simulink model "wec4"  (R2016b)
settings: Solver=ode4  StartTime=0  StopTime=1000  FixedStep=0.005  MaxStep=0.005  RelTol=1e-3  EnableMultiTasking=on
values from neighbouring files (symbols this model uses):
  arAdaptiveLawData = 1/2*zModelSimple.zModelPto.arFreq.*     zModelSimple.zModelPto.arMagnitude./     cos(zModelSimple.zModelPto.arPhase*pi/180+pi/2)    [IMPACT_Control.m]
  arAdaptiveLawDataX = 1/2*zModelSimpleX.zModelPto.arFreq.*         zModelSimpleX.zModelPto.arMagnitude./         cos(zModelSimpleX.zModelPto.arPhase*pi/180+pi/2)    [IMPACT_Control.m]
  arControllerRampGain = [0,0,1,1]    [IMPACT_Control.m]
  arControllerRampTime = [0 rStartRampTime rStartRampTime+rRampTimeLength 8000]    [IMPACT_Control.m]
  arEkfInitialisation = zeros(1,11)    [IMPACT_Control.m]
  arEkfInitialisationX = zeros(1,11)    [IMPACT_Control.m]
  arFrequency = zModelSimple.zModelPto.arFreq    [IMPACT_Control.m]
  arFrequencyRange = zModelSimple.zModelPto.arFreq    [IMPACT_Control.m]
  arFrequencyX = zModelSimpleX.zModelPto.arFreq    [IMPACT_Control.m]
  arImpedance = 1./zModelSimple.zModelPto.arMagnitude./zModelSimple.zModelPto.arFreq    [IMPACT_Control.m]
  arImpedanceX = 1./zModelSimpleX.zModelPto.arMagnitude./zModelSimpleX.zModelPto.arFreq    [IMPACT_Control.m]
  CentralPTOPreload = -1.6113e+07    (= -16113000)    [wecSimInputFile.m]
  F1 = [4.243 2.375 -12.243]    [wecSimInputFile.m]
  F2 = [4.243 -2.375 -12.243]    [wecSimInputFile.m]
  F3 = [-4.243 -2.375 -12.243]    [wecSimInputFile.m]
  F4 = [-4.243 2.375 -12.243]    [wecSimInputFile.m]
  FC = [0 0 -14]    [wecSimInputFile.m]
  iAdaptiveDamping = 0    [wec4IMPACT_Project.m]    (also in IMPACT_Control.m = handles.iAdaptiveDamping; wec1_IMPACT_Project.m; wec2_IMPACT_Project.m; wec3_IMPACT_Project.m)
  iControlType = 2    [wec4IMPACT_Project.m]    (also in IMPACT_Control.m = handles.iControlType; wec1_IMPACT_Project.m = 1; wec2_IMPACT_Project.m = 1; wec3_IMPACT_Project.m = 1)
  iPtoPositionConstraint = 1    [wec4IMPACT_Project.m]    (also in IMPACT_Control.m = handles.iPtoPositionConstraint; wec1_IMPACT_Project.m = 0; wec2_IMPACT_Project.m; wec3_IMPACT_Project.m)
  iSensorNoise = 0    [IMPACT_Control.m]
  m = m+1    (= 2)    [checkParamFile.m]
  PTOrotation = atan((T1(2)-F1(2))/(T1(1)-F1(1)))    [wecSimInputFile.m]
  rCogFloater = -8    [wec4_IMPACT_Model.m]    (also in paramInitial.m = get( handles.edit_rCogFloater, 'String' ); wec1_IMPACT_Model.m = -18; wec2_IMPACT_Model.m = -8.5; wec3_IMPACT_Model.m = -0.7)
  rCogSpar = -36.6    [wec4_IMPACT_Model.m]    (also in paramInitial.m = get( handles.edit_rCogSpar, 'String' ); wec3_IMPACT_Model.m = -21.3; wec3_IMPACT_Model2.m = -21.3)
  rDisplacementLimit = 10.000000    (= 10)    [wec4IMPACT_Project.m]    (also in IMPACT_Control.m = getValue(handles.edit_displacementLimit); wec1_IMPACT_Project.m; wec2_IMPACT_Project.m; wec3_IMPACT_Project.m = 3)
  rDisplacementLimitX = 10.000000    (= 10)    [wec4IMPACT_Project.m]    (also in IMPACT_Control.m = getValue(handles.edit_displacementLimitX); wec1_IMPACT_Project.m = 0; wec2_IMPACT_Project.m; wec3_IMPACT_Project.m = 0)
  rGainForAntiWIndUp = tfControllerDiscrete.rGain    [IMPACT_Control.m]
  rGainForAntiWIndUpX = tfControllerXDiscrete.rGain    [IMPACT_Control.m]
  rMaxForcePto = 300000000.000000    (= 300000000)    [wec4IMPACT_Project.m]    (also in IMPACT_Control.m = getValue(handles.edit_maxForcePto); wec1_IMPACT_Project.m = 1e+15; wec2_IMPACT_Project.m = 1e+15; wec3_IMPACT_Project.m = 1000000000)
  rMinForcePto = -300000000.000000    (= -300000000)    [wec4IMPACT_Project.m]    (also in IMPACT_Control.m = getValue(handles.edit_minForcePto); wec1_IMPACT_Project.m = -1e+15; wec2_IMPACT_Project.m = -1e+15; wec3_IMPACT_Project.m = -1000000000)
  rMooringX = 20000    [wec4_IMPACT_Model.m]    (also in paramInitial.m = get( handles.edit_rMooringX, 'String' ); wec3_IMPACT_Model.m = 10000; wec3_IMPACT_Model2.m = 10000)
  rMooringZ = 10000    [wec4_IMPACT_Model.m]    (also in paramInitial.m = get( handles.edit_rMooringZ, 'String' ); wec3_IMPACT_Model.m = 0; wec3_IMPACT_Model2.m = 0)
  rOutputSampleTime = 0.010000    (= 0.01)    [wec4IMPACT_Project.m]    (also in IMPACT_Control.m = getValue(handles.edit_outputSampleTime); wec1_IMPACT_Project.m; wec2_IMPACT_Project.m; wec3_IMPACT_Project.m)
  rPassiveDampingGain = -604830.000000    (= -604830)    [wec4IMPACT_Project.m]    (also in IMPACT_Control.m = getValue(handles.edit_gainPLD); wec1_IMPACT_Project.m = -214018.1537; wec2_IMPACT_Project.m = -1948070; wec3_IMPACT_Project.m = -519390)
  rPassiveDampingGainX = -278660.000000    (= -278660)    [wec4IMPACT_Project.m]    (also in IMPACT_Control.m = getValue(handles.edit_gainPLDX); wec1_IMPACT_Project.m = 0; wec2_IMPACT_Project.m = 0; wec3_IMPACT_Project.m = 0)
  rTetherPretension = 1.6113e+07    (= 16113000)    [wec4_IMPACT_Model.m]    (also in paramInitial.m = get( handles.edit_rTetherPretension, 'String' ); wec3_IMPACT_Model.m = 0; wec3_IMPACT_Model2.m = 0)
  rTetherSpring = 500000    [wec4_IMPACT_Model.m]    (also in paramInitial.m = get( handles.edit_rTetherSpring, 'String' ); wec3_IMPACT_Model.m = 0; wec3_IMPACT_Model2.m = 0)
  rUpperFrequencyLimit = EKFFloater.upperFreq    [IMPACT_Control.m]
  rXf = 4.243    [wec4AdditionalParams.m]
  rXs = 16.075    [wec4AdditionalParams.m]
  rYf = 2.375    [wec4AdditionalParams.m]
  rYs = 16.075    [wec4AdditionalParams.m]
  rZf = 4.243    [wec4AdditionalParams.m]
  rZs = 2.4350    (= 2.435)    [wec4AdditionalParams.m]
  rZTetherF = 6    [wec4AdditionalParams.m]
  rZTetherS = 2.4350    (= 2.435)    [wec4AdditionalParams.m]
  s = tf('s')    [wec4_IMPACT_Model.m]    (also in IMPACT_Control.m; wec1_IMPACT_Model.m; wec2_IMPACT_Model.m; wec3_IMPACT_Model.m)
  SidePTO1Preload = PreloadPTOCorner    (= 0)    [wecSimInputFile.m]
  SidePTO2Preload = PreloadPTOCorner    (= 0)    [wecSimInputFile.m]
  SidePTO3Preload = PreloadPTOCorner    (= 0)    [wecSimInputFile.m]
  SidePTO4Preload = PreloadPTOCorner    (= 0)    [wecSimInputFile.m]
  simu = simulationClass()    [wecSimInputFile.m]
  T1 = [16.075 16.075 -34.165]    [wecSimInputFile.m]
  T2 = [16.075 -16.075 -34.165]    [wecSimInputFile.m]
  T3 = [-16.075 -16.075 -34.165]    [wecSimInputFile.m]
  T4 = [-16.075 16.075 -34.165]    [wecSimInputFile.m]
  TC = [0 0 -34.165]    [wecSimInputFile.m]
  waves = waveClass('irregular')    [wecSimInputFile.m]
  Z = magPhaseToComplex(zModelTf)    [IMPACT_Control.m]
undefined symbols (not defined in the file or in its folder): arControllerDiscreteDen, arControllerDiscreteNum, arControllerDiscreteXDen, arControllerDiscreteXNum, arExcForceFloaterDen, arExcForceFloaterNum, arExcForceFloaterXDen, arExcForceFloaterXNum, arExcForceSparDen, arExcForceSparNum, arExcForceSparXDen, arExcForceSparXNum, arFexcFloaterDen, arFexcFloaterNum, arFexcFloaterXDen, arFexcFloaterXNum, arFexcSparDen, arFexcSparNum, arFexcSparXDen, arFexcSparXNum, Body, body, constraint, CTTime, deg, Elements, geometry, IRKB, kg, lenJ, mooring, N, pto, rAccelerationGainFloater, rAccelerationGainFloaterX, rAccelerationGainSpar, rAccelerationGainSparX, rad, rBuoyancyGainFloater, rBuoyancyGainFloaterX, rBuoyancyGainSpar, rBuoyancyGainSparX, rDampingGainFloater, rDampingGainFloaterX, rDampingGainSpar, rDampingGainSparX, Rigid, rMaxFocePto, wec4_float, wec4_reactor, WECSim_Lib, X, Y
libraries: nesl_utility x380, sm_lib x170, vrlib x91, simulink x12, WECSim_Lib x4
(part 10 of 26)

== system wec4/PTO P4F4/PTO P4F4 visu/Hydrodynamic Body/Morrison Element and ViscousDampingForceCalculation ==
  Displacement : Inport
  Acceleration : Inport  Port=2
  Velocity : Inport  Port=3
  Time : Inport  Port=4
  Abs1 : Abs
  Morrison Element Variant Subsystem : Subsystem  Variant=on
  Product : Product
  Product1 : Product  Multiplication=Matrix(*)
  Transport Delay : TransportDelay  DelayTime=10e-8
  "VisSum " : Sum  Inputs=+-
  "Viscous Damping Matrix (diagonal) " : Constant  Value=body.hydroForce.visDrag
  F_MorrisonAndViscous : Outport
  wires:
  Time/1 -> Morrison Element Variant Subsystem/4(time)
  Morrison Element Variant Subsystem/1(morison_force) -> "VisSum "/2
  Displacement/1 -> Morrison Element Variant Subsystem/1(displacement)
  Product/1 -> Product1/2  "v * |v|"
  "Viscous Damping Matrix (diagonal) "/1 -> Product1/1  "0.5 * cd * rho *A"
  Product1/1 -> "VisSum "/1
  Abs1/1 -> Product/2
  Acceleration/1 -> Transport Delay/1
  Transport Delay/1 -> Morrison Element Variant Subsystem/3(acceleration)
  "VisSum "/1 -> F_MorrisonAndViscous/1  "F_MorrisonAndViscous"
  Velocity/1 -> Abs1/1, Product/1, Morrison Element Variant Subsystem/2(velocity)

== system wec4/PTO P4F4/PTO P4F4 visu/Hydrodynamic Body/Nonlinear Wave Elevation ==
  Displacement : Inport
  Time : Inport  Port=2
  Add : Sum  Inputs=+-
  Center of Gravity : Constant  Value=body.cg
  Constant : Constant  Value=[0 0 0]
  Linear or Instantaneous Free Surface : Subsystem  Variant=on
  Mux : Mux  Inputs=2
  Wave Elevation : Outport
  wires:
  Time/1 -> Linear or Instantaneous Free Surface/2(In2)
  Constant/1 -> Mux/2
  Center of Gravity/1 -> Mux/1  "cg"
  Mux/1 -> Add/2
  Add/1 -> Linear or Instantaneous Free Surface/1(In1)  "x_cg"
  Linear or Instantaneous Free Surface/1(Out1) -> Wave Elevation/1
  Displacement/1 -> Add/1  "x"

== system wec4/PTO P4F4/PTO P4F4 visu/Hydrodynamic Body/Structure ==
  Total Force : Inport
  Body Properties : sm_lib/Body Elements/Solid  InertiaType=Custom  Mass=body.mass  MassUnits=kg  CenterOfMass=[0 0 0]  CenterOfMassUnits=m  MomentsOfInertia=body.momOfInertia  MomentsOfInertiaUnits=kg*m^2  ProductsOfInertia=[0 0 0]  ProductsOfInertiaUnits=kg*m^2  DensityBased=on  Density=1000  DensityUnits=kg/(m^3)  DoExposeReferenceFrame=on  SerializedFrames=<Frames/>  GraphicType=FromGeometry  MarkerShape=Sphere  MarkerSize=10  MarkerSizeUnits=m  GraphicVisPropType=SimpleVisualProperties  GraphicDiffuseColor=body.viz.color  GraphicSpecularColor=[0.5 0.5 0.5 1.0]  GraphicAmbientColor=[0.15 0.15 0.15 1.0]  GraphicEmissiveColor=[0.0 0.0 0.0 1.0]  GraphicShininess=75  GraphicOpacity=body.viz.opacity  GeometryShape=FromFile  RectangleSize=[1 1]  RectangleSizeUnits=m  BrickDimensions=[1 1 1]  BrickDimensionUnits=m  CylinderRadius=1  CylinderRadiusUnits=m  CylinderLength=1  CylinderLengthUnits=m  SphereRadius=1  SphereRadiusUnits=m  EllipsoidRadii=[1 1 1]  EllipsoidRadiiUnits=m  ExtrusionCrossSection=[1 1; -1 1; -1 -1; 1 -1]  ExtrusionCrossSectionUnits=m  ExtrusionLength=1  ExtrusionLengthUnits=m  PolygonNumSides=3  PolygonOuterRadius=1  PolygonOuterRadiusUnits=m  ExtGeomFileType=STL  ExtGeomFileName=.\geometry\pto_visu.stl  ExtGeomFileUnits=m  RevolutionCrossSection=[1 1; 1 -1; 2 -1; 2 1]  RevolutionCrossSectionUnits=m  RevolutionExtent=Full  RevolutionAngle=180  RevolutionAngleUnits=deg
  External Force and Torque : sm_lib/Forces and Torques/External Force and Torque  ForceResolutionFrame=World  EnableForceX=off  EnableForceY=off  EnableForceZ=off  EnableForce=on  TorqueResolutionFrame=World  EnableTorqueX=off  EnableTorqueY=off  EnableTorqueZ=off  EnableTorque=on
  Motion Sensor : Subsystem
  Rigid Transform (Setup CG) : sm_lib/Frames and Transforms/Rigid Transform  TranslationMethod=Cartesian  TranslationStandardOffset=0  TranslationLengthUnit=m  TranslationStandardAxis=+Z  TranslationCartesianOffset=body.cg  TranslationROffset=0  TranslationROffsetUnits=m  TranslationZOffset=0  TranslationZOffsetUnits=m  TranslationThetaOffset=0  TranslationThetaOffsetUnits=deg  RotationMethod=None  RotationAngleUnits=rad  RotationStandardAxis=+Y  RotationAngle=0.05  RotationArbitraryAxis=[0.57735026918962584 0.57735026918962584 0.57735026918962584]  FollAlignAxisA=+X  BaseAlignAxisA=+Y  FollAlignAxisB=+Y  BaseAlignAxisB=+Z  RotationSequenceAxes=FollowerAxes  RotationSequence=XYX  RotationSequenceAngles=[0 0 0]  RotationSequenceAnglesUnits=deg  RotationMatrix=[1 0 0; 0 1 0; 0 0 1]
  Rigid Transform (Setup Initial Disp) : sm_lib/Frames and Transforms/Rigid Transform  TranslationMethod=Cartesian  TranslationStandardOffset=0  TranslationLengthUnit=m  TranslationStandardAxis=+Z  TranslationCartesianOffset=body.initDisp.initLinDisp  TranslationROffset=0  TranslationROffsetUnits=m  TranslationZOffset=0  TranslationZOffsetUnits=m  TranslationThetaOffset=0  TranslationThetaOffsetUnits=deg  RotationMethod=ArbitraryAxis  RotationAngleUnits=rad  RotationStandardAxis=+Y  RotationAngle=body.initDisp.initAngularDispAngle  RotationArbitraryAxis=body.initDisp.initAngularDispAxis  FollAlignAxisA=+X  BaseAlignAxisA=+Y  FollAlignAxisB=+Y  BaseAlignAxisB=+Z  RotationSequenceAxes=FollowerAxes  RotationSequence=XYX  RotationSequenceAngles=[0 0 0]  RotationSequenceAnglesUnits=deg  RotationMatrix=[1 0 0; 0 1 0; 0 0 1]
  Selector : Selector  InputPortWidth=6  IndexOptions=Index vector (dialog)  Indices=[1:3]  OutputSizes=1
  Selector1 : Selector  InputPortWidth=6  IndexOptions=Index vector (dialog)  Indices=[4:6]  OutputSizes=1
  Simulink-PS Converter1 : nesl_utility/Simulink-PS Converter  PhysicalDomain=network_engine_domain  SubClassName=ps_input  LeftPortType=input  RightPortType=output  PseudoPeriodic=off  Frequencies=[]  NoiseDistribution=none  NoiseParameters=[]  Unit=1  AffineConversion=off  InputFiltering=off  SimscapeFilterOrder=1  InputFilterTimeConstant=0.001  UdotUserProvided=1
  Simulink-PS Converter2 : nesl_utility/Simulink-PS Converter  PhysicalDomain=network_engine_domain  SubClassName=ps_input  LeftPortType=input  RightPortType=output  PseudoPeriodic=off  Frequencies=[]  NoiseDistribution=none  NoiseParameters=[]  Unit=1  AffineConversion=off  InputFiltering=off  SimscapeFilterOrder=1  InputFilterTimeConstant=0.001  UdotUserProvided=1
  World Frame : sm_lib/Frames and Transforms/World Frame
  Conn Free Surface : PMIOPort  Port=1  Side=Right
  Response : Outport
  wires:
  Total Force/1 -> Selector1/1, Selector/1
  Selector/1 -> Simulink-PS Converter1/1
  Selector1/1 -> Simulink-PS Converter2/1
  Motion Sensor/1(Response) -> Response/1
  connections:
  External Force and Torque/LConn1 -- Simulink-PS Converter1/RConn1
  External Force and Torque/LConn2 -- Simulink-PS Converter2/RConn1
  Rigid Transform (Setup Initial Disp)/RConn1 -- Body Properties/RConn1 -- External Force and Torque/RConn1 -- Motion Sensor/RConn1
  Conn Free Surface/RConn1 -- Rigid Transform (Setup CG)/LConn1
  Rigid Transform (Setup Initial Disp)/LConn1 -- Rigid Transform (Setup CG)/RConn1
  World Frame/RConn1 -- Motion Sensor/LConn1

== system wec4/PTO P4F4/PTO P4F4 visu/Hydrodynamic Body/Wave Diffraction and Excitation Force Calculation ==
  Time : Inport
  Displacement : Inport  Port=2
  WaveElv : Inport  Port=3
  Add : Sum
  If2 : If  NumInputs=2  IfExpression=u1 < u2
  Linear Wave Excitation Force Variant Subsystem : Subsystem  Variant=on
  Merge1 : Merge
  No Ramp Function : Subsystem  TreatAsAtomicUnit=on
  Nonlinear FK Force Variant Subsystem : Subsystem  Variant=on
  Product : Product
  Ramp Function : Subsystem  TreatAsAtomicUnit=on
  Ramp Function Time : Constant  Value=simu.rampTime
  F_Excitation : Outport  PortDimensions=6
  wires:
  Nonlinear FK Force Variant Subsystem/1(Out1) -> Add/2
  Linear Wave Excitation Force Variant Subsystem/1(Out1) -> Add/1
  WaveElv/1 -> Nonlinear FK Force Variant Subsystem/3(In3)
  Displacement/1 -> Nonlinear FK Force Variant Subsystem/2(In2)
  Product/1 -> F_Excitation/1  "F_Excitation"
  Add/1 -> Product/2  "F_wave"
  Time/1 -> If2/1, Ramp Function/1(Time), Nonlinear FK Force Variant Subsystem/1(In1), Linear Wave Excitation Force Variant Subsystem/1(In1)
  Merge1/1 -> Product/1  "R"
  Ramp Function Time/1 -> If2/2
  If2/2 -> No Ramp Function/Action
  If2/1 -> Ramp Function/Action
  Ramp Function/1(R) -> Merge1/1
  No Ramp Function/1(R) -> Merge1/2

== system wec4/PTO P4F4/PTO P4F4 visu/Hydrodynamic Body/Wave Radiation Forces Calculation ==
  Velocity : Inport
  Acceleration : Inport  Port=2
  Time : Inport  Port=3
  Added Mass Matrix : Constant  Value=body.hydroForce.fAddedMass
  Product1 : Product  Multiplication=Matrix(*)
  SS CI and Constant-Damping-CoeVariant Subsystem : Subsystem  Variant=on
  Transport Delay : TransportDelay  DelayTime=10e-8
  F_RadiationDamping : Outport
  F_AddedMass : Outport  Port=2
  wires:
  Time/1 -> SS CI and Constant-Damping-CoeVariant Subsystem/2(In2)
  Acceleration/1 -> Transport Delay/1
  Transport Delay/1 -> Product1/2
  SS CI and Constant-Damping-CoeVariant Subsystem/1(Out1) -> F_RadiationDamping/1  "F_RadiationDamping"
  Velocity/1 -> SS CI and Constant-Damping-CoeVariant Subsystem/1(In1)
  Product1/1 -> F_AddedMass/1  "F_AddedMass"
  Added Mass Matrix/1 -> Product1/1

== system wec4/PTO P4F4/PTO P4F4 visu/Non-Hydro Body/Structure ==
  Total Force : Inport
  Body Properties : sm_lib/Body Elements/Solid  InertiaType=Custom  Mass=body.mass  MassUnits=kg  CenterOfMass=[0 0 0]  CenterOfMassUnits=m  MomentsOfInertia=body.momOfInertia  MomentsOfInertiaUnits=kg*m^2  ProductsOfInertia=[0 0 0]  ProductsOfInertiaUnits=kg*m^2  DensityBased=on  Density=1000  DensityUnits=kg/(m^3)  DoExposeReferenceFrame=on  SerializedFrames=<Frames/>  GraphicType=FromGeometry  MarkerShape=Sphere  MarkerSize=10  MarkerSizeUnits=m  GraphicVisPropType=SimpleVisualProperties  GraphicDiffuseColor=body.viz.color  GraphicSpecularColor=[0.5 0.5 0.5 1.0]  GraphicAmbientColor=[0.15 0.15 0.15 1.0]  GraphicEmissiveColor=[0.0 0.0 0.0 1.0]  GraphicShininess=75  GraphicOpacity=body.viz.opacity  GeometryShape=FromFile  RectangleSize=[1 1]  RectangleSizeUnits=m  BrickDimensions=[1 1 1]  BrickDimensionUnits=m  CylinderRadius=1  CylinderRadiusUnits=m  CylinderLength=1  CylinderLengthUnits=m  SphereRadius=1  SphereRadiusUnits=m  EllipsoidRadii=[1 1 1]  EllipsoidRadiiUnits=m  ExtrusionCrossSection=[1 1; -1 1; -1 -1; 1 -1]  ExtrusionCrossSectionUnits=m  ExtrusionLength=1  ExtrusionLengthUnits=m  PolygonNumSides=3  PolygonOuterRadius=1  PolygonOuterRadiusUnits=m  ExtGeomFileType=STL  ExtGeomFileName=.\geometry\pto_visu.stl  ExtGeomFileUnits=m  RevolutionCrossSection=[1 1; 1 -1; 2 -1; 2 1]  RevolutionCrossSectionUnits=m  RevolutionExtent=Full  RevolutionAngle=180  RevolutionAngleUnits=deg
  External Force and Torque : sm_lib/Forces and Torques/External Force and Torque  ForceResolutionFrame=World  EnableForceX=off  EnableForceY=off  EnableForceZ=off  EnableForce=on  TorqueResolutionFrame=World  EnableTorqueX=off  EnableTorqueY=off  EnableTorqueZ=off  EnableTorque=on
  Motion Sensor : Subsystem
  Rigid Transform (Setup CG) : sm_lib/Frames and Transforms/Rigid Transform  TranslationMethod=Cartesian  TranslationStandardOffset=0  TranslationLengthUnit=m  TranslationStandardAxis=+Z  TranslationCartesianOffset=body.cg  TranslationROffset=0  TranslationROffsetUnits=m  TranslationZOffset=0  TranslationZOffsetUnits=m  TranslationThetaOffset=0  TranslationThetaOffsetUnits=deg  RotationMethod=None  RotationAngleUnits=rad  RotationStandardAxis=+Y  RotationAngle=0.05  RotationArbitraryAxis=[0.57735026918962584 0.57735026918962584 0.57735026918962584]  FollAlignAxisA=+X  BaseAlignAxisA=+Y  FollAlignAxisB=+Y  BaseAlignAxisB=+Z  RotationSequenceAxes=FollowerAxes  RotationSequence=XYX  RotationSequenceAngles=[0 0 0]  RotationSequenceAnglesUnits=deg  RotationMatrix=[1 0 0; 0 1 0; 0 0 1]
  Rigid Transform (Setup Initial Disp) : sm_lib/Frames and Transforms/Rigid Transform  TranslationMethod=Cartesian  TranslationStandardOffset=0  TranslationLengthUnit=m  TranslationStandardAxis=+Z  TranslationCartesianOffset=body.initDisp.initLinDisp  TranslationROffset=0  TranslationROffsetUnits=m  TranslationZOffset=0  TranslationZOffsetUnits=m  TranslationThetaOffset=0  TranslationThetaOffsetUnits=deg  RotationMethod=ArbitraryAxis  RotationAngleUnits=rad  RotationStandardAxis=+Y  RotationAngle=body.initDisp.initAngularDispAngle  RotationArbitraryAxis=body.initDisp.initAngularDispAxis  FollAlignAxisA=+X  BaseAlignAxisA=+Y  FollAlignAxisB=+Y  BaseAlignAxisB=+Z  RotationSequenceAxes=FollowerAxes  RotationSequence=XYX  RotationSequenceAngles=[0 0 0]  RotationSequenceAnglesUnits=deg  RotationMatrix=[1 0 0; 0 1 0; 0 0 1]
  Selector : Selector  InputPortWidth=6  IndexOptions=Index vector (dialog)  Indices=[1:3]  OutputSizes=1
  Selector1 : Selector  InputPortWidth=6  IndexOptions=Index vector (dialog)  Indices=[4:6]  OutputSizes=1
  Simulink-PS Converter1 : nesl_utility/Simulink-PS Converter  PhysicalDomain=network_engine_domain  SubClassName=ps_input  LeftPortType=input  RightPortType=output  PseudoPeriodic=off  Frequencies=[]  NoiseDistribution=none  NoiseParameters=[]  Unit=1  AffineConversion=off  InputFiltering=off  SimscapeFilterOrder=1  InputFilterTimeConstant=0.001  UdotUserProvided=1
  Simulink-PS Converter2 : nesl_utility/Simulink-PS Converter  PhysicalDomain=network_engine_domain  SubClassName=ps_input  LeftPortType=input  RightPortType=output  PseudoPeriodic=off  Frequencies=[]  NoiseDistribution=none  NoiseParameters=[]  Unit=1  AffineConversion=off  InputFiltering=off  SimscapeFilterOrder=1  InputFilterTimeConstant=0.001  UdotUserProvided=1
  World Frame : sm_lib/Frames and Transforms/World Frame
  Conn Free Surface : PMIOPort  Port=1  Side=Right
  Response : Outport
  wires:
  Total Force/1 -> Selector1/1, Selector/1
  Selector/1 -> Simulink-PS Converter1/1
  Selector1/1 -> Simulink-PS Converter2/1
  Motion Sensor/1(Response) -> Response/1
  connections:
  External Force and Torque/LConn1 -- Simulink-PS Converter1/RConn1
  External Force and Torque/LConn2 -- Simulink-PS Converter2/RConn1
  Rigid Transform (Setup Initial Disp)/RConn1 -- Body Properties/RConn1 -- External Force and Torque/RConn1 -- Motion Sensor/RConn1
  Conn Free Surface/RConn1 -- Rigid Transform (Setup CG)/LConn1
  Rigid Transform (Setup Initial Disp)/LConn1 -- Rigid Transform (Setup CG)/RConn1
  World Frame/RConn1 -- Motion Sensor/LConn1

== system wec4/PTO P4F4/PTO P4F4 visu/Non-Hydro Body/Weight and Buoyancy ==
  Add1 : Sum  Inputs=+-
  Assignment (Add Net Bouyancy Force to Z-Direction) : Assignment  IndexOptions=Index vector (dialog)  Indices=3  OutputSizes=1
  Body Mass : Constant  Value=body.mass
  Constant1 : Constant  Value=[0 0 0 0 0 0]
  Gravity : Constant  Value=simu.g
  Product : Product
  Product1 : Product  Inputs=3
  Volume : Constant  Value=body.dispVol
  Water Density : Constant  Value=simu.rho
  Out1 : Outport
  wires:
  Add1/1 -> Assignment (Add Net Bouyancy Force to Z-Direction)/2
  Product1/1 -> Add1/2  "F_Buoyancy"
  Product/1 -> Add1/1  "F_Gravity"
  Water Density/1 -> Product1/1  "rho"
  Gravity/1 -> Product/1, Product1/2  "g"
  Volume/1 -> Product1/3  "Vol"
  Assignment (Add Net Bouyancy Force to Z-Direction)/1 -> Out1/1  "F_Restoring"
  Constant1/1 -> Assignment (Add Net Bouyancy Force to Z-Direction)/1
  Body Mass/1 -> Product/2  "m"

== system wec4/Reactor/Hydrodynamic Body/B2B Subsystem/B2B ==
  CrossCoupling : Subsystem
  vel : Outport
  acc : Outport  Port=2
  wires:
  CrossCoupling/2(acc) -> acc/1
  CrossCoupling/1(vel) -> vel/1

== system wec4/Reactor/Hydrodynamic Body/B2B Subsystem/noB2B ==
  vel_in : Inport
  acc_in : Inport  Port=2
  vel : Outport
  acc : Outport  Port=2
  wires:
  acc_in/1 -> acc/1
  vel_in/1 -> vel/1  "x"

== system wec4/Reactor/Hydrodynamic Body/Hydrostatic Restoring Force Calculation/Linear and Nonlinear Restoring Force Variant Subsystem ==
  note: 1) Add Subsystem or Model blocks as valid variant choices. 2) You cannot connect blocks at this level. At simulation, connectivity is automatically determined, based on the active variant and port name matching.
  In1 : Inport
  In2 : Inport  Port=2
  "Linear Hydrostatic Restoring Force " : Subsystem  VariantControl=sv_linearHydro
  Nonlinear Hydrostatic Restoring Force : Subsystem  VariantControl=sv_nonlinearHydro
  Out1 : Outport

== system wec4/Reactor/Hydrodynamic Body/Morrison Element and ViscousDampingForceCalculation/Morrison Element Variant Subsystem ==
  note: 1) Add Subsystem or Model blocks as valid variant choices. 2) You cannot connect blocks at this level. At simulation, connectivity is automatically determined, based on the active variant and port name matching.
  displacement : Inport
  velocity : Inport  Port=2
  acceleration : Inport  Port=3
  time : Inport  Port=4
  Morrison Element Off : Subsystem  VariantControl=sv_MEOff
  Morrison Element On : Subsystem  Variant=on  VariantControl=sv_MEOn
  morison_force : Outport

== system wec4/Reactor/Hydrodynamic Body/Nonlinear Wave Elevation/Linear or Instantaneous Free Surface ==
  note: 1) Add Subsystem or Model blocks as valid variant choices. 2) You cannot connect blocks at this level. At simulation, connectivity is automatically determined, based on the active variant and port name matching.
  In1 : Inport
  In2 : Inport  Port=2
  "Instantaneous Water Free Surface  " : Subsystem  VariantControl=sv_instFS
  "Mean Water Free Surface " : Subsystem  VariantControl=sv_meanFS
  Out1 : Outport

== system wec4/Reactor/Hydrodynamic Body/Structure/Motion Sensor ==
  note: Measures the position, velocity, and acceleration of the follower (F) frame relative to the base (B) frame. Ouputs a bus of 3 signals, each signal is a vector length 6.
  Angle : MATLAB Function  TreatAsAtomicUnit=on
  Bus Creator : BusCreator  Inputs=3
  Mux : Mux
  Mux1 : Mux  Inputs=6
  Mux2 : Mux  Inputs=6
  PS-Simulink Converter{,1..15} (16 alike) : nesl_utility/PS-Simulink Converter  PhysicalDomain=network_engine_domain  SubClassName=ps_output  LeftPortType=input  RightPortType=output  PseudoPeriodic=off  Frequencies=[]  Unit=1  AffineConversion=off
  Transform Sensor : sm_lib/Frames and Transforms/Transform Sensor  MeasurementFrame=World  SenseAngle=off  SenseAxis=off  SenseAngle1=off  SenseAngle2=off  SenseAngle3=off  SenseQ=on  SenseR=off  SenseOmegaX=on  SenseOmegaY=on  SenseOmegaZ=on  SenseOmega1=off  SenseOmega2=off  SenseOmega3=off  SenseQDot=off  SenseRDot=off  SenseAlphaX=on  SenseAlphaY=on  SenseAlphaZ=on  SenseAlpha1=off  SenseAlpha2=off  SenseAlpha3=off  SenseQDDot=off  SenseRDDot=off  SenseX=on  SenseY=on  SenseZ=on  SenseRad=off  SenseAzim=off  SenseDist=off  SenseInc=off  SenseXDot=on  SenseYDot=on  SenseZDot=on  SenseRadDot=off  SenseAzimDot=off  SenseDistDot=off  SenseIncDot=off  SenseXDDot=on  SenseYDDot=on  SenseZDDot=on  SenseRadDDot=off  SenseAzimDDot=off  SenseDistDDot=off  SenseIncDDot=off
  F : PMIOPort  Port=1  Side=Right
  B : PMIOPort  Port=2  Side=Left
  Response : Outport
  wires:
  PS-Simulink Converter/1 -> Angle/1(Q)
  PS-Simulink Converter4/1 -> Mux2/4  "alphax"
  PS-Simulink Converter10/1 -> Mux1/1  "vx"
  PS-Simulink Converter12/1 -> Mux1/3  "vz"
  PS-Simulink Converter13/1 -> Mux2/1  "ax"
  PS-Simulink Converter14/1 -> Mux2/2  "ay"
  Mux/1 -> Bus Creator/1  "disp"
  Mux1/1 -> Bus Creator/2  "vel"
  Mux2/1 -> Bus Creator/3  "acc"
  Angle/1(E) -> Mux/4
  PS-Simulink Converter7/1 -> Mux/1  "x"
  PS-Simulink Converter8/1 -> Mux/2  "y"
  PS-Simulink Converter9/1 -> Mux/3  "z"
  PS-Simulink Converter5/1 -> Mux2/5  "alphay"
  PS-Simulink Converter6/1 -> Mux2/6  "alphaz"
  PS-Simulink Converter1/1 -> Mux1/4  "omegax"
  PS-Simulink Converter2/1 -> Mux1/5  "omegay"
  PS-Simulink Converter11/1 -> Mux1/2  "vy"
  PS-Simulink Converter3/1 -> Mux1/6  "omegaz"
  PS-Simulink Converter15/1 -> Mux2/3  "az"
  Bus Creator/1 -> Response/1
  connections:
  Transform Sensor/RConn1 -- F/RConn1
  B/RConn1 -- Transform Sensor/LConn1
  Transform Sensor/RConn2 -- PS-Simulink Converter/LConn1
  PS-Simulink Converter15/LConn1 -- Transform Sensor/RConn17
  PS-Simulink Converter14/LConn1 -- Transform Sensor/RConn16
  PS-Simulink Converter13/LConn1 -- Transform Sensor/RConn15
  PS-Simulink Converter12/LConn1 -- Transform Sensor/RConn14
  PS-Simulink Converter11/LConn1 -- Transform Sensor/RConn13
  PS-Simulink Converter10/LConn1 -- Transform Sensor/RConn12
  PS-Simulink Converter9/LConn1 -- Transform Sensor/RConn11
  PS-Simulink Converter8/LConn1 -- Transform Sensor/RConn10
  PS-Simulink Converter7/LConn1 -- Transform Sensor/RConn9
  PS-Simulink Converter4/LConn1 -- Transform Sensor/RConn6
  PS-Simulink Converter5/LConn1 -- Transform Sensor/RConn7
  PS-Simulink Converter6/LConn1 -- Transform Sensor/RConn8
  PS-Simulink Converter1/LConn1 -- Transform Sensor/RConn3
  PS-Simulink Converter2/LConn1 -- Transform Sensor/RConn4
  PS-Simulink Converter3/LConn1 -- Transform Sensor/RConn5

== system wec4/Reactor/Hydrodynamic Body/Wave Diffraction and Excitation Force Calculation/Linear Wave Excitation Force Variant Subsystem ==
  note: 1) Add Subsystem or Model blocks as valid variant choices. 2) You cannot connect blocks at this level. At simulation, connectivity is automatically determined, based on the active variant and port name matching.
  In1 : Inport
  Irregular Wave Excitation Force : Subsystem  VariantControl=sv_irregularWaves
  No Wave Excitation Force : Subsystem  VariantControl=sv_noWave
  Regular Wave Excitation Force : Subsystem  VariantControl=sv_regularWaves
  User Defined Wave Excitation Force : Subsystem  VariantControl=sv_udfWaves
  Out1 : Outport

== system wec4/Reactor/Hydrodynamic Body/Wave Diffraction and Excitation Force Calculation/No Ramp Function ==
  Action Port : ActionPort  ActionType=else
  Constant : Constant
  R : Outport  InitialOutput=1
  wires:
  Constant/1 -> R/1

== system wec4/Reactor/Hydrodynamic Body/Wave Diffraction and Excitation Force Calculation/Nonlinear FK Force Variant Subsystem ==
  note: 1) Add Subsystem or Model blocks as valid variant choices. 2) You cannot connect blocks at this level. At simulation, connectivity is automatically determined, based on the active variant and port name matching.
  In1 : Inport
  In2 : Inport  Port=2
  In3 : Inport  Port=3
  No Nonlinear FroudeKrylov Force : Subsystem  VariantControl=sv_linearHydro
  With Nonlinear FroudeKrylov Force : Subsystem  TreatAsAtomicUnit=on  SystemSampleTime=simu.dtNL  VariantControl=sv_nonlinearHydro
  Out1 : Outport

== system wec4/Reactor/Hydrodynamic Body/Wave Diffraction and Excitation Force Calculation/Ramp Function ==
  Time : Inport
  Action Port : ActionPort  ActionType=then
  Add : Sum
  Add1 : Sum
  Constant : Constant  Value=1/2
  Constant1 : Constant
  Constant2 : Constant  Value=3*pi/2
  Constant3 : Constant  Value=pi
  Divide : Product  Inputs=*/
  Product : Product
  Product1 : Product
  Ramp Time : Constant  Value=simu.rampTime
  Sine Wave Function : Sin  TimeSource=Use external signal  SampleTime=0
  R : Outport
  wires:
  Divide/1 -> Product1/2  "frequency"
  Constant3/1 -> Divide/1
  Product1/1 -> Add1/1
  Add1/1 -> Sine Wave Function/1
  Constant2/1 -> Add1/2  "phase"
  Ramp Time/1 -> Divide/2  "t_ramp"
  Time/1 -> Product1/1  "t"
  Product/1 -> R/1
  Constant/1 -> Product/2
  Constant1/1 -> Add/1
  Sine Wave Function/1 -> Add/2
  Add/1 -> Product/1

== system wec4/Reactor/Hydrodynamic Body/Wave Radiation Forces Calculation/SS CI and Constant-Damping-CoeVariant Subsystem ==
  note: 1) Add Subsystem or Model blocks as valid variant choices. 2) You cannot connect blocks at this level. At simulation, connectivity is automatically determined, based on the active variant and port name matching.
  In1 : Inport
  In2 : Inport  Port=2
  Constant Coefficients : Subsystem  VariantControl=sv_constantCoeff
  Convolution Integral Calculation : Subsystem  VariantControl=sv_convolution
  "State-Space Calculation " : Subsystem  VariantControl=sv_stateSpace
  Out1 : Outport

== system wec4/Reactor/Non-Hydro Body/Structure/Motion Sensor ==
  note: Measures the position, velocity, and acceleration of the follower (F) frame relative to the base (B) frame. Ouputs a bus of 3 signals, each signal is a vector length 6.
  Angle : MATLAB Function  TreatAsAtomicUnit=on
  Bus Creator : BusCreator  Inputs=3
  Mux : Mux
  Mux1 : Mux  Inputs=6
  Mux2 : Mux  Inputs=6
  PS-Simulink Converter{,1..15} (16 alike) : nesl_utility/PS-Simulink Converter  PhysicalDomain=network_engine_domain  SubClassName=ps_output  LeftPortType=input  RightPortType=output  PseudoPeriodic=off  Frequencies=[]  Unit=1  AffineConversion=off
  Transform Sensor : sm_lib/Frames and Transforms/Transform Sensor  MeasurementFrame=World  SenseAngle=off  SenseAxis=off  SenseAngle1=off  SenseAngle2=off  SenseAngle3=off  SenseQ=on  SenseR=off  SenseOmegaX=on  SenseOmegaY=on  SenseOmegaZ=on  SenseOmega1=off  SenseOmega2=off  SenseOmega3=off  SenseQDot=off  SenseRDot=off  SenseAlphaX=on  SenseAlphaY=on  SenseAlphaZ=on  SenseAlpha1=off  SenseAlpha2=off  SenseAlpha3=off  SenseQDDot=off  SenseRDDot=off  SenseX=on  SenseY=on  SenseZ=on  SenseRad=off  SenseAzim=off  SenseDist=off  SenseInc=off  SenseXDot=on  SenseYDot=on  SenseZDot=on  SenseRadDot=off  SenseAzimDot=off  SenseDistDot=off  SenseIncDot=off  SenseXDDot=on  SenseYDDot=on  SenseZDDot=on  SenseRadDDot=off  SenseAzimDDot=off  SenseDistDDot=off  SenseIncDDot=off
  F : PMIOPort  Port=1  Side=Right
  B : PMIOPort  Port=2  Side=Left
  Response : Outport
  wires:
  PS-Simulink Converter/1 -> Angle/1(Q)
  PS-Simulink Converter4/1 -> Mux2/4  "alphax"
  PS-Simulink Converter10/1 -> Mux1/1  "vx"
  PS-Simulink Converter12/1 -> Mux1/3  "vz"
  PS-Simulink Converter13/1 -> Mux2/1  "ax"
  PS-Simulink Converter14/1 -> Mux2/2  "ay"
  Mux/1 -> Bus Creator/1  "disp"
  Mux1/1 -> Bus Creator/2  "vel"
  Mux2/1 -> Bus Creator/3  "acc"
  Angle/1(E) -> Mux/4
  PS-Simulink Converter7/1 -> Mux/1  "x"
  PS-Simulink Converter8/1 -> Mux/2  "y"
  PS-Simulink Converter9/1 -> Mux/3  "z"
  PS-Simulink Converter5/1 -> Mux2/5  "alphay"
  PS-Simulink Converter6/1 -> Mux2/6  "alphaz"
  PS-Simulink Converter1/1 -> Mux1/4  "omegax"
  PS-Simulink Converter2/1 -> Mux1/5  "omegay"
  PS-Simulink Converter11/1 -> Mux1/2  "vy"
  PS-Simulink Converter3/1 -> Mux1/6  "omegaz"
  PS-Simulink Converter15/1 -> Mux2/3  "az"
  Bus Creator/1 -> Response/1
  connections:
  Transform Sensor/RConn1 -- F/RConn1
  B/RConn1 -- Transform Sensor/LConn1
  Transform Sensor/RConn2 -- PS-Simulink Converter/LConn1
  PS-Simulink Converter15/LConn1 -- Transform Sensor/RConn17
  PS-Simulink Converter14/LConn1 -- Transform Sensor/RConn16
  PS-Simulink Converter13/LConn1 -- Transform Sensor/RConn15
  PS-Simulink Converter12/LConn1 -- Transform Sensor/RConn14
  PS-Simulink Converter11/LConn1 -- Transform Sensor/RConn13
  PS-Simulink Converter10/LConn1 -- Transform Sensor/RConn12
  PS-Simulink Converter9/LConn1 -- Transform Sensor/RConn11
  PS-Simulink Converter8/LConn1 -- Transform Sensor/RConn10
  PS-Simulink Converter7/LConn1 -- Transform Sensor/RConn9
  PS-Simulink Converter4/LConn1 -- Transform Sensor/RConn6
  PS-Simulink Converter5/LConn1 -- Transform Sensor/RConn7
  PS-Simulink Converter6/LConn1 -- Transform Sensor/RConn8
  PS-Simulink Converter1/LConn1 -- Transform Sensor/RConn3
  PS-Simulink Converter2/LConn1 -- Transform Sensor/RConn4
  PS-Simulink Converter3/LConn1 -- Transform Sensor/RConn5

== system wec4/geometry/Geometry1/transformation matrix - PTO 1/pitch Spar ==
  Xs : Inport
  Phi : Inport  Port=2
  Zs : Inport  Port=3
  Product{20..23} (4 alike) : Product
  Sum10 : Sum  Inputs=+-
  Sum11 : Sum
  Trigonometric Function10 : Trigonometry
  Trigonometric Function11 : Trigonometry  Operator=cos
  d_xs_phi : Outport
  d_zs_phi : Outport  Port=2
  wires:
  Sum10/1 -> d_xs_phi/1
  Trigonometric Function10/1 -> Product23/1, Product20/1
  Phi/1 -> Trigonometric Function10/1, Trigonometric Function11/1
  Xs/1 -> Product20/2, Product22/1
  Product20/1 -> Sum11/2
  Product21/1 -> Sum11/1
  Product23/1 -> Sum10/2
  Trigonometric Function11/1 -> Product21/2, Product22/2
  Product22/1 -> Sum10/1
  Zs/1 -> Product23/2, Product21/1
  Sum11/1 -> d_zs_phi/1

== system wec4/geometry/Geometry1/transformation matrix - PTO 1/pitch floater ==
  x_f : Inport
  phiF : Inport  Port=2
  z_f : Inport  Port=3
  Product{16..19} (4 alike) : Product
  Sum8 : Sum
  Sum9 : Sum  Inputs=+-
  Trigonometric Function8 : Trigonometry
  Trigonometric Function9 : Trigonometry  Operator=cos
  d_xf_phi : Outport
  d_zf_phi : Outport  Port=2
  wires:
  x_f/1 -> Product16/2, Product18/1
  Sum8/1 -> d_xf_phi/1  "d_xf_phi"
  Trigonometric Function8/1 -> Product16/1, Product19/1
  phiF/1 -> Trigonometric Function9/1, Trigonometric Function8/1
  Product17/1 -> Sum9/1
  Trigonometric Function9/1 -> Product18/2, Product17/2
  Product18/1 -> Sum8/1
  Product19/1 -> Sum8/2
  Product16/1 -> Sum9/2
  Sum9/1 -> d_zf_phi/1  "d_zf_phi"
  z_f/1 -> Product17/1, Product19/2

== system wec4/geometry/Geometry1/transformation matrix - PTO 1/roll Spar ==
  y_s : Inport
  theta : Inport  Port=2
  z_s : Inport  Port=3
  Product{8..11} (4 alike) : Product
  Sum4 : Sum
  Sum5 : Sum  Inputs=+-
  Trigonometric Function4 : Trigonometry
  Trigonometric Function5 : Trigonometry  Operator=cos
  d_ys_theta : Outport
  d_zs_theta : Outport  Port=2
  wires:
  theta/1 -> Trigonometric Function4/1, Trigonometric Function5/1
  Product8/1 -> Sum4/1
  Product9/1 -> Sum4/2
  Product10/1 -> Sum5/2
  z_s/1 -> Product9/2, Product11/1
  Sum4/1 -> d_ys_theta/1  "d_ys_theta"
  Trigonometric Function4/1 -> Product10/1, Product9/1
  Product11/1 -> Sum5/1
  Sum5/1 -> d_zs_theta/1  "d_zs_theta"
  Trigonometric Function5/1 -> Product8/2, Product11/2
  y_s/1 -> Product8/1, Product10/2

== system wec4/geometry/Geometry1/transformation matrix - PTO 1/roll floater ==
  y_f : Inport
  thetaF : Inport  Port=2
  z_f : Inport  Port=3
  Product{12..15} (4 alike) : Product
  Sum6 : Sum  Inputs=+-
  Sum7 : Sum
  Trigonometric Function6 : Trigonometry
  Trigonometric Function7 : Trigonometry  Operator=cos
  d_yf_theta : Outport
  d_zf_theta : Outport  Port=2
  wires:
  y_f/1 -> Product14/1, Product12/2
  z_f/1 -> Product15/2, Product13/1
  Trigonometric Function6/1 -> Product15/1, Product12/1
  Product12/1 -> Sum7/2
  Product15/1 -> Sum6/2
  Sum6/1 -> d_yf_theta/1  "d_yf_theta"
  Product13/1 -> Sum7/1
  Product14/1 -> Sum6/1
  Trigonometric Function7/1 -> Product13/2, Product14/2
  thetaF/1 -> Trigonometric Function6/1, Trigonometric Function7/1
  Sum7/1 -> d_zf_theta/1  "d_zf_theta"

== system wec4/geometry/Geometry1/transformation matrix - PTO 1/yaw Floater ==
  x_f : Inport
  psiF : Inport  Port=2
  y_f : Inport  Port=3
  Product{2..3,6..7} (4 alike) : Product
  Sum1 : Sum
  Sum3 : Sum  Inputs=+-
  Trigonometric Function1 : Trigonometry
  Trigonometric Function3 : Trigonometry  Operator=cos
  d_xf_psi : Outport
  d_yf_psi : Outport  Port=2
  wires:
  Product3/1 -> Sum1/2
  Product2/1 -> Sum1/1
  psiF/1 -> Trigonometric Function1/1, Trigonometric Function3/1
  Sum3/1 -> d_yf_psi/1  "d_ys_psi"
  Product6/1 -> Sum3/1
  Trigonometric Function3/1 -> Product6/2, Product2/2
  Product7/1 -> Sum3/2
  Sum1/1 -> d_xf_psi/1  "d_xf_Psi"
  y_f/1 -> Product3/2, Product6/1
  Trigonometric Function1/1 -> Product7/1, Product3/1
  x_f/1 -> Product7/2, Product2/1

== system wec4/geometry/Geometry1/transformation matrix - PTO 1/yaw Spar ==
  Xs : Inport
  PsiS : Inport  Port=2
  Ys : Inport  Port=3
  Product{,1,4..5} (4 alike) : Product
  Sum : Sum
  Sum2 : Sum  Inputs=+-
  Trigonometric Function : Trigonometry
  Trigonometric Function2 : Trigonometry  Operator=cos
  d_xs_psi : Outport
  d_ys_psi : Outport  Port=2
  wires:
  Product1/1 -> Sum/2
  Xs/1 -> Product/1, Product5/2
  Sum2/1 -> d_ys_psi/1  "d_ys_psi"
  Trigonometric Function2/1 -> Product/2, Product4/2
  PsiS/1 -> Trigonometric Function/1, Trigonometric Function2/1
  Sum/1 -> d_xs_psi/1  "d_xs_psi"
  Product/1 -> Sum/1
  Product5/1 -> Sum2/2
  Trigonometric Function/1 -> Product1/1, Product5/1
  Product4/1 -> Sum2/1
  Ys/1 -> Product1/2, Product4/1

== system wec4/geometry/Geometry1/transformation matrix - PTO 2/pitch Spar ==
  Xs : Inport
  Phi : Inport  Port=2
  Zs : Inport  Port=3
  Product{20..23} (4 alike) : Product
  Sum10 : Sum  Inputs=+-
  Sum11 : Sum
  Trigonometric Function10 : Trigonometry
  Trigonometric Function11 : Trigonometry  Operator=cos
  d_xs_phi : Outport
  d_zs_phi : Outport  Port=2
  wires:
  Sum11/1 -> d_zs_phi/1
  Zs/1 -> Product21/1, Product23/2
  Product22/1 -> Sum10/1
  Trigonometric Function11/1 -> Product22/2, Product21/2
  Product23/1 -> Sum10/2
  Product21/1 -> Sum11/1
  Product20/1 -> Sum11/2
  Xs/1 -> Product22/1, Product20/2
  Phi/1 -> Trigonometric Function11/1, Trigonometric Function10/1
  Trigonometric Function10/1 -> Product20/1, Product23/1
  Sum10/1 -> d_xs_phi/1

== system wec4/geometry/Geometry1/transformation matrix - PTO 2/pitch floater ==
  x_f : Inport
  phiF : Inport  Port=2
  z_f : Inport  Port=3
  Product{16..19} (4 alike) : Product
  Sum8 : Sum
  Sum9 : Sum  Inputs=+-
  Trigonometric Function8 : Trigonometry
  Trigonometric Function9 : Trigonometry  Operator=cos
  d_xf_phi : Outport
  d_zf_phi : Outport  Port=2
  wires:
  z_f/1 -> Product19/2, Product17/1
  Sum9/1 -> d_zf_phi/1  "d_zf_phi"
  Product16/1 -> Sum9/2
  Product19/1 -> Sum8/2
  Product18/1 -> Sum8/1
  Trigonometric Function9/1 -> Product17/2, Product18/2
  Product17/1 -> Sum9/1
  phiF/1 -> Trigonometric Function8/1, Trigonometric Function9/1
  Trigonometric Function8/1 -> Product19/1, Product16/1
  Sum8/1 -> d_xf_phi/1  "d_xf_phi"
  x_f/1 -> Product18/1, Product16/2

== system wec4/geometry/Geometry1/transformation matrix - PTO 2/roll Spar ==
  y_s : Inport
  theta : Inport  Port=2
  z_s : Inport  Port=3
  Product{8..11} (4 alike) : Product
  Sum4 : Sum
  Sum5 : Sum  Inputs=+-
  Trigonometric Function4 : Trigonometry
  Trigonometric Function5 : Trigonometry  Operator=cos
  d_ys_theta : Outport
  d_zs_theta : Outport  Port=2
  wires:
  y_s/1 -> Product10/2, Product8/1
  Trigonometric Function5/1 -> Product11/2, Product8/2
  Sum5/1 -> d_zs_theta/1  "d_zs_theta"
  Product11/1 -> Sum5/1
  Trigonometric Function4/1 -> Product9/1, Product10/1
  Sum4/1 -> d_ys_theta/1  "d_ys_theta"
  z_s/1 -> Product11/1, Product9/2
  Product10/1 -> Sum5/2
  Product9/1 -> Sum4/2
  Product8/1 -> Sum4/1
  theta/1 -> Trigonometric Function5/1, Trigonometric Function4/1

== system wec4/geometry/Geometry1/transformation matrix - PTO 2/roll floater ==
  y_f : Inport
  thetaF : Inport  Port=2
  z_f : Inport  Port=3
  Product{12..15} (4 alike) : Product
  Sum6 : Sum  Inputs=+-
  Sum7 : Sum
  Trigonometric Function6 : Trigonometry
  Trigonometric Function7 : Trigonometry  Operator=cos
  d_yf_theta : Outport
  d_zf_theta : Outport  Port=2
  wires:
  Sum7/1 -> d_zf_theta/1  "d_zf_theta"
  thetaF/1 -> Trigonometric Function7/1, Trigonometric Function6/1
  Trigonometric Function7/1 -> Product14/2, Product13/2
  Product14/1 -> Sum6/1
  Product13/1 -> Sum7/1
  Sum6/1 -> d_yf_theta/1  "d_yf_theta"
  Product15/1 -> Sum6/2
  Product12/1 -> Sum7/2
  Trigonometric Function6/1 -> Product12/1, Product15/1
  z_f/1 -> Product13/1, Product15/2
  y_f/1 -> Product12/2, Product14/1

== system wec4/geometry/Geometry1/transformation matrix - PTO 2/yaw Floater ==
  x_f : Inport
  psiF : Inport  Port=2
  y_f : Inport  Port=3
  Product{2..3,6..7} (4 alike) : Product
  Sum1 : Sum
  Sum3 : Sum  Inputs=+-
  Trigonometric Function1 : Trigonometry
  Trigonometric Function3 : Trigonometry  Operator=cos
  d_xf_psi : Outport
  d_yf_psi : Outport  Port=2
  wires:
  x_f/1 -> Product2/1, Product7/2
  Trigonometric Function1/1 -> Product3/1, Product7/1
  y_f/1 -> Product6/1, Product3/2
  Sum1/1 -> d_xf_psi/1  "d_xf_Psi"
  Product7/1 -> Sum3/2
  Trigonometric Function3/1 -> Product2/2, Product6/2
  Product6/1 -> Sum3/1
  Sum3/1 -> d_yf_psi/1  "d_ys_psi"
  psiF/1 -> Trigonometric Function3/1, Trigonometric Function1/1
  Product2/1 -> Sum1/1
  Product3/1 -> Sum1/2

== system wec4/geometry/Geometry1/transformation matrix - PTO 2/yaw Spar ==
  Xs : Inport
  PsiS : Inport  Port=2
  Ys : Inport  Port=3
  Product{,1,4..5} (4 alike) : Product
  Sum : Sum
  Sum2 : Sum  Inputs=+-
  Trigonometric Function : Trigonometry
  Trigonometric Function2 : Trigonometry  Operator=cos
  d_xs_psi : Outport
  d_ys_psi : Outport  Port=2
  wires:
  Ys/1 -> Product4/1, Product1/2
  Product4/1 -> Sum2/1
  Trigonometric Function/1 -> Product5/1, Product1/1
  Product5/1 -> Sum2/2
  Product/1 -> Sum/1
  Sum/1 -> d_xs_psi/1  "d_xs_psi"
  PsiS/1 -> Trigonometric Function2/1, Trigonometric Function/1
  Trigonometric Function2/1 -> Product4/2, Product/2
  Sum2/1 -> d_ys_psi/1  "d_ys_psi"
  Xs/1 -> Product5/2, Product/1
  Product1/1 -> Sum/2

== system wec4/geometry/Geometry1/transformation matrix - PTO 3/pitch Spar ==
  Xs : Inport
  Phi : Inport  Port=2
  Zs : Inport  Port=3
  Product{20..23} (4 alike) : Product
  Sum10 : Sum  Inputs=+-
  Sum11 : Sum
  Trigonometric Function10 : Trigonometry
  Trigonometric Function11 : Trigonometry  Operator=cos
  d_xs_phi : Outport
  d_zs_phi : Outport  Port=2
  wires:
  Sum11/1 -> d_zs_phi/1
  Zs/1 -> Product21/1, Product23/2
  Product22/1 -> Sum10/1
  Trigonometric Function11/1 -> Product22/2, Product21/2
  Product23/1 -> Sum10/2
  Product21/1 -> Sum11/1
  Product20/1 -> Sum11/2
  Xs/1 -> Product22/1, Product20/2
  Phi/1 -> Trigonometric Function11/1, Trigonometric Function10/1
  Trigonometric Function10/1 -> Product20/1, Product23/1
  Sum10/1 -> d_xs_phi/1

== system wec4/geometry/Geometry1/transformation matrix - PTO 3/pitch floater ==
  x_f : Inport
  phiF : Inport  Port=2
  z_f : Inport  Port=3
  Product{16..19} (4 alike) : Product
  Sum8 : Sum
  Sum9 : Sum  Inputs=+-
  Trigonometric Function8 : Trigonometry
  Trigonometric Function9 : Trigonometry  Operator=cos
  d_xf_phi : Outport
  d_zf_phi : Outport  Port=2
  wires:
  z_f/1 -> Product19/2, Product17/1
  Sum9/1 -> d_zf_phi/1  "d_zf_phi"
  Product16/1 -> Sum9/2
  Product19/1 -> Sum8/2
  Product18/1 -> Sum8/1
  Trigonometric Function9/1 -> Product17/2, Product18/2
  Product17/1 -> Sum9/1
  phiF/1 -> Trigonometric Function8/1, Trigonometric Function9/1
  Trigonometric Function8/1 -> Product19/1, Product16/1
  Sum8/1 -> d_xf_phi/1  "d_xf_phi"
  x_f/1 -> Product18/1, Product16/2

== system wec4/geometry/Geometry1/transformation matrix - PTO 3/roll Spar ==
  y_s : Inport
  theta : Inport  Port=2
  z_s : Inport  Port=3
  Product{8..11} (4 alike) : Product
  Sum4 : Sum
  Sum5 : Sum  Inputs=+-
  Trigonometric Function4 : Trigonometry
  Trigonometric Function5 : Trigonometry  Operator=cos
  d_ys_theta : Outport
  d_zs_theta : Outport  Port=2
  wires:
  y_s/1 -> Product10/2, Product8/1
  Trigonometric Function5/1 -> Product11/2, Product8/2
  Sum5/1 -> d_zs_theta/1  "d_zs_theta"
  Product11/1 -> Sum5/1
  Trigonometric Function4/1 -> Product9/1, Product10/1
  Sum4/1 -> d_ys_theta/1  "d_ys_theta"
  z_s/1 -> Product11/1, Product9/2
  Product10/1 -> Sum5/2
  Product9/1 -> Sum4/2
  Product8/1 -> Sum4/1
  theta/1 -> Trigonometric Function5/1, Trigonometric Function4/1

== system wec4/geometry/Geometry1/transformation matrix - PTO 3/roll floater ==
  y_f : Inport
  thetaF : Inport  Port=2
  z_f : Inport  Port=3
  Product{12..15} (4 alike) : Product
  Sum6 : Sum  Inputs=+-
  Sum7 : Sum
  Trigonometric Function6 : Trigonometry
  Trigonometric Function7 : Trigonometry  Operator=cos
  d_yf_theta : Outport
  d_zf_theta : Outport  Port=2
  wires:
  Sum7/1 -> d_zf_theta/1  "d_zf_theta"
  thetaF/1 -> Trigonometric Function7/1, Trigonometric Function6/1
  Trigonometric Function7/1 -> Product14/2, Product13/2
  Product14/1 -> Sum6/1
  Product13/1 -> Sum7/1
  Sum6/1 -> d_yf_theta/1  "d_yf_theta"
  Product15/1 -> Sum6/2
  Product12/1 -> Sum7/2
  Trigonometric Function6/1 -> Product12/1, Product15/1
  z_f/1 -> Product13/1, Product15/2
  y_f/1 -> Product12/2, Product14/1

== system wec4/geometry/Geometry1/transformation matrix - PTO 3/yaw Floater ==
  x_f : Inport
  psiF : Inport  Port=2
  y_f : Inport  Port=3
  Product{2..3,6..7} (4 alike) : Product
  Sum1 : Sum
  Sum3 : Sum  Inputs=+-
  Trigonometric Function1 : Trigonometry
  Trigonometric Function3 : Trigonometry  Operator=cos
  d_xf_psi : Outport
  d_yf_psi : Outport  Port=2
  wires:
  x_f/1 -> Product2/1, Product7/2
  Trigonometric Function1/1 -> Product3/1, Product7/1
  y_f/1 -> Product6/1, Product3/2
  Sum1/1 -> d_xf_psi/1  "d_xf_Psi"
  Product7/1 -> Sum3/2
  Trigonometric Function3/1 -> Product2/2, Product6/2
  Product6/1 -> Sum3/1
  Sum3/1 -> d_yf_psi/1  "d_ys_psi"
  psiF/1 -> Trigonometric Function3/1, Trigonometric Function1/1
  Product2/1 -> Sum1/1
  Product3/1 -> Sum1/2

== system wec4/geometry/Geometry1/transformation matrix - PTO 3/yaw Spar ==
  Xs : Inport
  PsiS : Inport  Port=2
  Ys : Inport  Port=3
  Product{,1,4..5} (4 alike) : Product
  Sum : Sum
  Sum2 : Sum  Inputs=+-
  Trigonometric Function : Trigonometry
  Trigonometric Function2 : Trigonometry  Operator=cos
  d_xs_psi : Outport
  d_ys_psi : Outport  Port=2
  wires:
  Ys/1 -> Product4/1, Product1/2
  Product4/1 -> Sum2/1
  Trigonometric Function/1 -> Product5/1, Product1/1
  Product5/1 -> Sum2/2
  Product/1 -> Sum/1
  Sum/1 -> d_xs_psi/1  "d_xs_psi"
  PsiS/1 -> Trigonometric Function2/1, Trigonometric Function/1
  Trigonometric Function2/1 -> Product4/2, Product/2
  Sum2/1 -> d_ys_psi/1  "d_ys_psi"
  Xs/1 -> Product5/2, Product/1
  Product1/1 -> Sum/2

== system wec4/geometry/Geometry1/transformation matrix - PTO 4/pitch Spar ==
  Xs : Inport
  Phi : Inport  Port=2
  Zs : Inport  Port=3
  Product{20..23} (4 alike) : Product
  Sum10 : Sum  Inputs=+-
  Sum11 : Sum
  Trigonometric Function10 : Trigonometry
  Trigonometric Function11 : Trigonometry  Operator=cos
  d_xs_phi : Outport
  d_zs_phi : Outport  Port=2
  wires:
  Sum11/1 -> d_zs_phi/1
  Zs/1 -> Product21/1, Product23/2
  Product22/1 -> Sum10/1
  Trigonometric Function11/1 -> Product22/2, Product21/2
  Product23/1 -> Sum10/2
  Product21/1 -> Sum11/1
  Product20/1 -> Sum11/2
  Xs/1 -> Product22/1, Product20/2
  Phi/1 -> Trigonometric Function11/1, Trigonometric Function10/1
  Trigonometric Function10/1 -> Product20/1, Product23/1
  Sum10/1 -> d_xs_phi/1
